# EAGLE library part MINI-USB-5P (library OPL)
SMD Mini USB
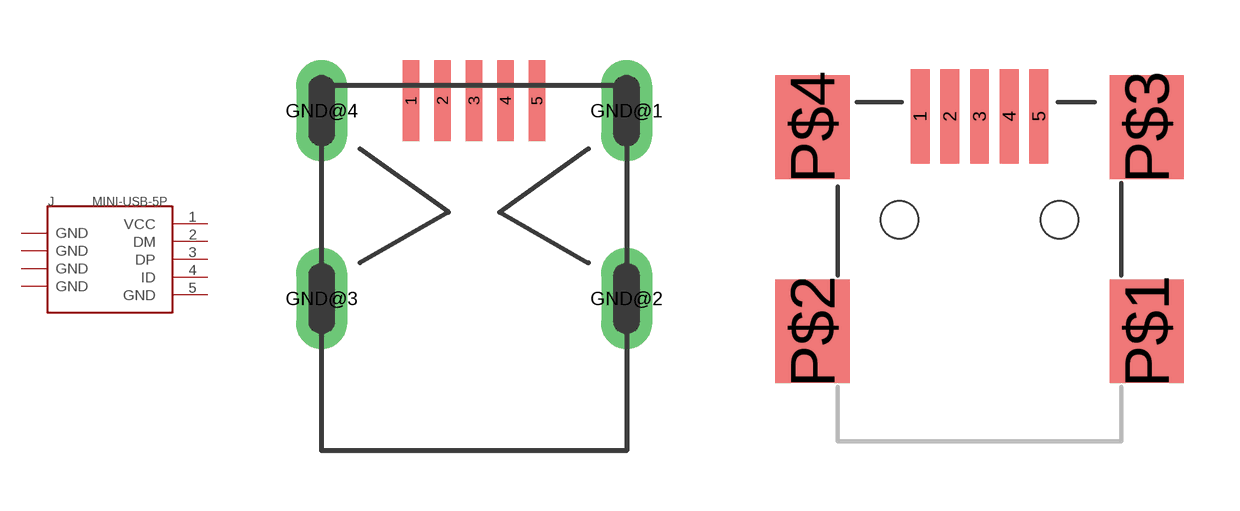
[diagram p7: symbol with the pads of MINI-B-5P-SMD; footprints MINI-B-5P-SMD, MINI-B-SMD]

Designator prefix J

## MINI-USB-5P-3400030P1  [MINI-B-5P-SMD]
1  VCC
2  DM
3  DP
4  ID
5  GND
GND@1  GND
GND@2  GND
GND@3  GND
GND@4  GND

## MINI-USB-5P-3400020P1  [MINI-B-SMD]
1  VCC
2  DM
3  DP
4  ID
5  GND
P$1  GND
P$2  GND
P$3  GND
P$4  GND

## Footprint MINI-B-5P-SMD (pad centres in mm)
smd 0.406 x 2.032: 1 -1.575,4.191; 2 -0.787,4.191; 3 0,4.191; 4 0.787,4.191; 5 1.575,4.191
drill 0.635 pad 1.27 long: GND@1 3.81,3.937; GND@2 3.81,-0.762; GND@3 -3.81,-0.762; GND@4 -3.81,3.937

## Footprint MINI-B-SMD (pad centres in mm)
USB Series Mini-B Surface Mounted
smd 0.508 x 2.54: 1 -1.6,4.191; 2 -0.8,4.191; 3 0,4.191; 4 0.8,4.191; 5 1.6,4.191
smd 2 x 2.794: P$1 4.5,-1.603; P$2 -4.5,-1.603; P$3 4.5,3.897; P$4 -4.5,3.897
hole 1.016 at -2.159,1.397
hole 1.016 at 2.159,1.397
